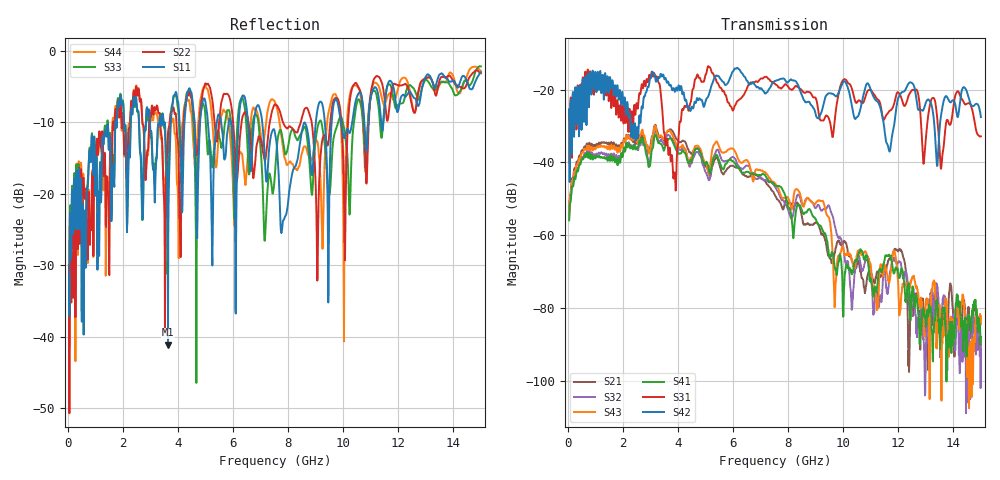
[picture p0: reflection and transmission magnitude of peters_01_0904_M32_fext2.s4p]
# MHZ S RI R 50.00
! FREQ  S11  S12  S13  S14
!  S21  S22  S23  S24
!  S31  S32  S33  S34
!  S41  S42  S43  S44
!  REAL  IMAG  REAL  IMAG  REAL  IMAG  REAL  IMAG
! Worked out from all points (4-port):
!   1496 points, 50 MHz to 15 GHz, reference 50 ohm
!   strongest paths, dB at 50 MHz, 3.79 GHz, 7.53 GHz, 11.27 GHz, 15 GHz:
!     S42: -25.4, -20.1, -17.6, -23.5, -27.6
!     S31: -25.6, -38.5, -18.5, -22.8, -32.8
!     S41: -55.9, -34.0, -46.3, -71.3, -87.9
!     S43: -54.3, -32.3, -45.8, -79.0, -82.1
!     S32: -55.4, -33.5, -46.8, -78.4, -88.0
!     S21: -53.4, -31.3, -49.1, -70.1, -89.9
!   lowest |S11| = -41.1 dB at 3.64 GHz (marker M1), VSWR 1.02, Z = 49.2 + j0.29 ohm
!   |S11| at or under -10 dB: start of sweep to 1.733 GHz; 7.061 GHz to 9.007 GHz (1.946 GHz wide, 24.2 % of centre); 9.916 GHz to 10.33 GHz (412.7 MHz wide, 4.08 % of centre)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
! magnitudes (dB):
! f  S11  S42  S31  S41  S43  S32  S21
! 50 MHz  -31.4  -25.4  -25.6  -55.9  -54.3  -55.4  -53.4
! 3.1 GHz  -16.6  -15.3  -16.5  -35.7  -32.5  -34.3  -32.2
! 3.64 GHz  -41.1  -17.8  -36.2  -33.8  -31.2  -32.4  -31.5
! 5.13 GHz  -12.2  -21.3  -13.8  -42.2  -43.2  -44.9  -43.4
! 9.06 GHz  -8.4  -27.8  -24.0  -56.6  -50.7  -51.9  -56.6
! 9.7 GHz  -6.9  -21.7  -27.9  -69.0  -78.6  -57.6  -64.7
! 15 GHz  -3.0  -27.6  -32.8  -87.9  -82.1  -88.0  -89.9
